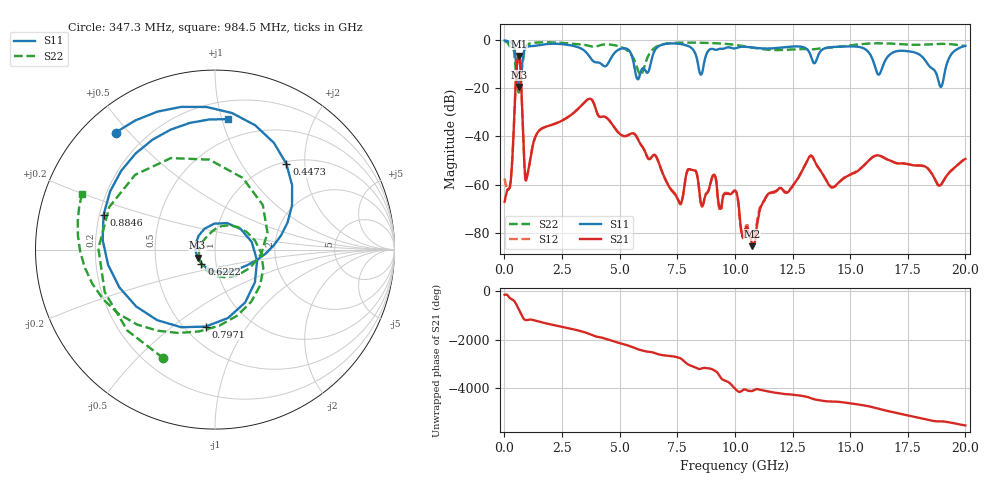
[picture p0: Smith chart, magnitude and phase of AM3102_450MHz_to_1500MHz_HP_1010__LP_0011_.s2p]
!Agilent Technologies,E8364B,MY43040894,A.07.50.67
!Agilent E8364B: A.07.50.67
!Date: Thursday, January 11, 2018 06:10:31
!Correction: S11(Full 2 Port(1,2))
!S21(Full 2 Port(1,2))
!S12(Full 2 Port(1,2))
!S22(Full 2 Port(1,2))
!S2P File: Measurements: S11, S21, S12, S22:
# Hz S  dB  R 50
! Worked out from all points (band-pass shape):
!   1601 points, 10 MHz to 20 GHz, reference 50 ohm
!   highest |S21| = -6.52 dB at 622.2 MHz (marker M1); lowest = -85.6 dB at 10.74 GHz (marker M2)
!   |S21| within 3 dB of the highest: 553.4 MHz to 680.1 MHz (126.7 MHz wide, 20.5 % of centre)
!   lowest |S11| = -19.4 dB at 634.7 MHz (marker M3), VSWR 1.24, Z = 41 - j3.79 ohm
!   |S11| at or under -10 dB: 5.619 GHz to 6.341 GHz (721.3 MHz wide, 12.1 % of centre); 16.05 GHz to 16.45 GHz (400 MHz wide, 2.46 % of centre); 18.38 GHz to 19.19 GHz (812 MHz wide, 4.32 % of centre)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
!   |S22| runs from -21.7 to -0.3 dB; largest |S21 - S12| = 0.0016
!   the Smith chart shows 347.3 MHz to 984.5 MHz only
!   S11 on the Smith chart (normalised r, x): 347.3 MHz: 0.09, +0.46; 447.3 MHz: 1.04, +1.62; 622.2 MHz: 0.85, -0.13; 797.1 MHz: 0.63, -0.66; 884.6 MHz: 0.22, +0.15; 984.5 MHz: 0.34, +1.05
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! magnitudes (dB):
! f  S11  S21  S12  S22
! 10 MHz  -0.1  -67.2  -57.5  -0.3
! 347.3 MHz  -1.4  -48.9  -48.8  -3.5
! 447.3 MHz  -4.1  -26.9  -26.9  -7.4
! 622.2 MHz  -19.3  -6.5  -6.5  -21.7
! 634.7 MHz  -19.4  -6.7  -6.7  -21.7
! 797.1 MHz  -7.3  -36.1  -36.1  -9.0
! 884.6 MHz  -3.7  -54.4  -54.6  -3.8
! 984.5 MHz  -2.7  -56.5  -56.8  -1.9
! 1.484 GHz  -2.1  -37.8  -37.9  -0.9
! 3.346 GHz  -3.5  -27.1  -27.1  -1.7
! 5.795 GHz  -16.2  -41.2  -41.2  -12.4
! 6.682 GHz  -2.6  -50.5  -50.5  -2.2
! 7.619 GHz  -1.5  -67.8  -68.1  -1.0
! 8.043 GHz  -2.7  -53.6  -53.7  -0.9
! 8.581 GHz  -13.5  -68.9  -69.2  -1.0
! 10.01 GHz  -3.4  -62.6  -62.5  -1.9
! 10.74 GHz  -3.0  -85.6  -82.8  -3.0
! 13.34 GHz  -7.8  -48.2  -48.2  -3.8
! 14.24 GHz  -2.8  -61.2  -61.2  -3.0
! 16.68 GHz  -6.3  -49.8  -49.8  -1.3
! 18.94 GHz  -19.4  -60.1  -60.3  -1.5
! 20 GHz  -2.3  -49.3  -49.5  -2.4
